FUNCTION_BLOCK FB_DO_IED_LD1_ATCC1_TapPos EXTENDS FB_AcsiCommonControllableDataClass
VAR_INPUT
	valWTr: FB_AcsiDATypeValWithTrans := (fc:=ACSI_FC_ST, TrgOp:=ACSI_TrgOp_dchg, bLinkResult:=THIS^.AddDataToContainer(ipData:=valWTr));
	q: FB_AcsiDATypeQuality := (fc:=ACSI_FC_ST, TrgOp:=ACSI_TrgOp_qchg, bLinkResult:=THIS^.AddDataToContainer(ipData:=q));
	t: FB_AcsiDATypeTimeStamp := (fc:=ACSI_FC_ST, bLinkResult:=THIS^.AddDataToContainer(ipData:=t));
	stSeld: FB_AcsiBATypeBOOLEAN := (fc:=ACSI_FC_ST, TrgOp:=ACSI_TrgOp_dchg, bLinkResult:=THIS^.AddDataToContainer(ipData:=stSeld));
	ctlModel: FB_AcsiDATypeCtlModels := (fc:=ACSI_FC_CF, TrgOp:=ACSI_TrgOp_dchg, eValue:=E_AcsiCtlModels.DirectWithEnhancedSecurity, bLinkResult:=THIS^.AddDataToContainer(ipData:=ctlModel));
	Oper: FB_AcsiCDC_Oper_INT8 := (fc:=ACSI_FC_CO, bLinkResult:=THIS^.AddDataToContainer(ipData:=Oper));
	
	fbControl: FB_DirectControl := (ipCtrl:=THIS^.AddServerJob(ipEvent:=fbControl, ipCompletion:=fbControl), eType:=E_AcsiCDCType.ISC, ipBehVal:=fbIED.IEDLD1.ATCC1.Beh.stVal);
END_VAR
VAR
END_VAR

END_FUNCTION_BLOCK
